PROGRAM ModbusRTU_Master
VAR
	ModbusRtuMaster	: ModbusRtuMasterV2_Generic;
	Timeout			: TIME:=T#1S;
	Data_01			: WORD;
	Data_02			: WORD;
	Data_03			: ARRAY[1..10] OF WORD;
	Data_04			: ARRAY[1..10] OF WORD;	
	Data_05			: WORD:=1;	 
	Data_06			: WORD:=666;
	Data_07			: DWORD:=3;
	Data_08			: ARRAY[1..100] OF WORD:=[100(1)];
	
	step		: INT;
	Start		: BOOL;
	i			: INT;
	ErrMsg_01: Tc2_ModbusRTU.MODBUS_ERRORS;
	ErrMsg_02: Tc2_ModbusRTU.MODBUS_ERRORS;
	ErrMsg_03: Tc2_ModbusRTU.MODBUS_ERRORS;
	ErrMsg_04: Tc2_ModbusRTU.MODBUS_ERRORS;
	ErrMsg_05: Tc2_ModbusRTU.MODBUS_ERRORS;
	ErrMsg_06: Tc2_ModbusRTU.MODBUS_ERRORS;
	ErrMsg_07: Tc2_ModbusRTU.MODBUS_ERRORS;
	ErrMsg_08: Tc2_ModbusRTU.MODBUS_ERRORS;
	ErrCount_01: INT;
	ErrCount_02: INT;
	ErrCount_03: INT;
	ErrCount_04: INT;
	ErrCount_05: INT;
	ErrCount_06: INT;
	ErrCount_07: INT;
	ErrCount_08: INT;
	ResetErrCount: BOOL;
	Counter: INT;
END_VAR

IF ResetErrCount THEN
	ErrCount_01:=0;
	ErrCount_02:=0;
	ErrCount_03:=0;
	ErrCount_04:=0;
	ErrCount_05:=0;
	ErrCount_06:=0;
	ErrCount_07:=0;
	ErrCount_08:=0;
	ResetErrCount:=FALSE;
END_IF
CASE step OF 
0: 
IF Start THEN
	step:=8;
	Counter:=Counter+1;	
//	Start:=FALSE;
END_IF
1:
// 读取线圈，对应Modsim中 01:Coil Status
	ModbusRtuMaster.ReadCoils(
		UnitID:=1 , 
		Quantity:=10 , 
		MBAddr:=0 , 	// 起始地址0，对应Modsim中地址00001——00010
		cbLength:=SIZEOF(Data_01) , // 读取10个bit，放在一个word中，占用2个字节 , 
		pMemoryAddr:=ADR(Data_01) , 
		AuxQuantity:= , 
		AuxMBAddr:= , 
		AuxcbLength:= , 
		pAuxMemoryAddr:= , 
		Execute:=TRUE , 
		Timeout:=Timeout , 
		RxBuffer:=RxBuffer , 
		TxBuffer:=TxBuffer , 
		BUSY=> , 
		Error=> , 
		ErrorId=> , 
		cbRead=> );
	IF NOT ModbusRtuMaster.BUSY THEN
		ModbusRtuMaster.ReadCoils(	Execute:=FALSE , RxBuffer:=RxBuffer , TxBuffer:=TxBuffer );
		step:=step+1;
		IF ModbusRtuMaster.Error THEN
			ErrMsg_01:=ModbusRtuMaster.ErrorId;
			ErrCount_01:=ErrCount_01+1;
		END_IF
	END_IF
2:
// 读取输入状态，对应Modsim中 02:Input Status
	ModbusRtuMaster.ReadInputStatus(
	UnitID:=1 , 
	Quantity:=10 , 	// 读取10个bit状态
	MBAddr:=0 , 	// 起始地址0，对应Modsim中地址10001——10010
	cbLength:=SIZEOF(Data_02) , // 读取10个bit，放在一个word中，占用2个字节
	pMemoryAddr:=ADR(Data_02) , 
	AuxQuantity:= , 
	AuxMBAddr:= , 
	AuxcbLength:= , 
	pAuxMemoryAddr:= , 
	Execute:=TRUE , 
	Timeout:=Timeout , 
	RxBuffer:=RxBuffer , 
	TxBuffer:=TxBuffer , 
	BUSY=> , 
	Error=> , 
	ErrorId=> , 
	cbRead=> );
	IF NOT ModbusRtuMaster.BUSY THEN
		ModbusRtuMaster.ReadInputStatus(	Execute:=FALSE , RxBuffer:=RxBuffer , TxBuffer:=TxBuffer );
		step:=step+1;
		IF ModbusRtuMaster.Error THEN
			ErrMsg_02:=ModbusRtuMaster.ErrorId;
			ErrCount_02:=ErrCount_02+1;
		END_IF
	END_IF
3:
// 读取保持寄存器，对应Modsim中 03:Holding Registers
	ModbusRtuMaster.ReadRegs(
	UnitID:=1 , 
	Quantity:=10 , 	// 读取10个寄存器数值，20个BYTE
	MBAddr:=0 , 	// 起始地址，0对应Modsim中地址40001——40010
	cbLength:=SIZEOF(Data_03) , // 读取10个寄存器，放在一个数组中，占用20个字节
	pMemoryAddr:=ADR(Data_03) , 
	AuxQuantity:= , 
	AuxMBAddr:= , 
	AuxcbLength:= , 
	pAuxMemoryAddr:= , 
	Execute:=TRUE , 
	Timeout:=Timeout , 
	RxBuffer:=RxBuffer , 
	TxBuffer:=TxBuffer , 
	BUSY=> , 
	Error=> , 
	ErrorId=> , 
	cbRead=> );
	IF NOT ModbusRtuMaster.BUSY THEN
		ModbusRtuMaster.ReadRegs(	Execute:=FALSE , RxBuffer:=RxBuffer , TxBuffer:=TxBuffer );
		step:=step+1;
		IF ModbusRtuMaster.Error THEN
			ErrMsg_03:=ModbusRtuMaster.ErrorId;
			ErrCount_03:=ErrCount_03+1;
		END_IF
	END_IF
4:
// 读取输入寄存器，对应Modsim中 04:Input Registers
	ModbusRtuMaster.ReadInputRegs(
	UnitID:=1 , 
	Quantity:=10 , 	// 读取10个寄存器数值，20个BYTE
	MBAddr:=0 , 	// 起始地址，0对应Modsim中地址30001——30010
	cbLength:=SIZEOF(Data_04) , // 读取10个寄存器，放在一个数组中，占用20个字节
	pMemoryAddr:=ADR(Data_04) , 
	AuxQuantity:= , 
	AuxMBAddr:= , 
	AuxcbLength:= , 
	pAuxMemoryAddr:= , 
	Execute:=TRUE , 
	Timeout:=Timeout , 
	RxBuffer:=RxBuffer , 
	TxBuffer:=TxBuffer , 
	BUSY=> , 
	Error=> , 
	ErrorId=> , 
	cbRead=> );
	IF NOT ModbusRtuMaster.BUSY THEN
		ModbusRtuMaster.ReadInputRegs(	Execute:=FALSE , RxBuffer:=RxBuffer , TxBuffer:=TxBuffer );
		step:=step+1;
		IF ModbusRtuMaster.Error THEN
			ErrMsg_04:=ModbusRtuMaster.ErrorId;
			ErrCount_04:=ErrCount_04+1;
		END_IF
		Data_05.0:=NOT Data_05.0;
	END_IF
5:
// 写入单个线圈Force Single Coil，对应Modsim中 01:Coil Status
	ModbusRtuMaster.WriteSingleCoil(
	UnitID:=1 , 
	Quantity:=1 , 	// 写入1个bit
	MBAddr:=50 , 	// 起始地址，50对应Modsim中地址00051
	cbLength:=SIZEOF(Data_05) , 
	pMemoryAddr:=ADR(Data_05) , 
	AuxQuantity:= , 
	AuxMBAddr:= , 
	AuxcbLength:= , 
	pAuxMemoryAddr:= , 
	Execute:=TRUE , 
	Timeout:=Timeout , 
	RxBuffer:=RxBuffer , 
	TxBuffer:=TxBuffer , 
	BUSY=> , 
	Error=> , 
	ErrorId=> , 
	cbRead=> );
	IF NOT ModbusRtuMaster.BUSY THEN
		ModbusRtuMaster.WriteSingleCoil(	Execute:=FALSE , RxBuffer:=RxBuffer , TxBuffer:=TxBuffer );
		step:=step+1;
		IF ModbusRtuMaster.Error THEN
			ErrMsg_05:=ModbusRtuMaster.ErrorId;
			ErrCount_05:=ErrCount_05+1;
		END_IF
		Data_06:=Data_06+1;
	END_IF
6:
// 写入单个寄存器Preset Single Register，对应Modsim中 03:Holding Registers
	ModbusRtuMaster.WriteSingleRegister(
	UnitID:=1 , 
	Quantity:=1 , 	// 写入1个寄存器，2个Byte
	MBAddr:=50 , 	// 起始地址，50对应Modsim中地址40051
	cbLength:=SIZEOF(Data_06) , 
	pMemoryAddr:=ADR(Data_06) , 
	AuxQuantity:= , 
	AuxMBAddr:= , 
	AuxcbLength:= , 
	pAuxMemoryAddr:= , 
	Execute:=TRUE , 
	Timeout:=Timeout , 
	RxBuffer:=RxBuffer , 
	TxBuffer:=TxBuffer , 
	BUSY=> , 
	Error=> , 
	ErrorId=> , 
	cbRead=> );
	IF NOT ModbusRtuMaster.BUSY THEN
		ModbusRtuMaster.WriteSingleRegister(	Execute:=FALSE , RxBuffer:=RxBuffer , TxBuffer:=TxBuffer );
		step:=step+1;
		IF ModbusRtuMaster.Error THEN
			ErrMsg_06:=ModbusRtuMaster.ErrorId;
			ErrCount_06:=ErrCount_06+1;
		END_IF
		Data_07:=ROL(Data_07,1);
	END_IF
7:
// 写入多个线圈Force Multiple Coils，对应Modsim中 01:Coil Status
	ModbusRtuMaster.WriteMultipleCoils(
	UnitID:=1 , 
	Quantity:=20 , 	// 写入20个bit
	MBAddr:=80 , 	// 起始地址，80对应Modsim中地址00081——00100
	cbLength:=SIZEOF(Data_07) , 	// 数据来自一个DWORD
	pMemoryAddr:=ADR(Data_07) , 
	AuxQuantity:= , 
	AuxMBAddr:= , 
	AuxcbLength:= , 
	pAuxMemoryAddr:= , 
	Execute:=TRUE , 
	Timeout:=Timeout , 
	RxBuffer:=RxBuffer , 
	TxBuffer:=TxBuffer , 
	BUSY=> , 
	Error=> , 
	ErrorId=> , 
	cbRead=> );
	IF NOT ModbusRtuMaster.BUSY THEN
		ModbusRtuMaster.WriteMultipleCoils(	Execute:=FALSE , RxBuffer:=RxBuffer , TxBuffer:=TxBuffer );
		step:=step+1;
		IF ModbusRtuMaster.Error THEN
			ErrMsg_07:=ModbusRtuMaster.ErrorId;
			ErrCount_07:=ErrCount_07+1;
		END_IF
		FOR i:=1 TO 20 DO
			Data_08[i]:=Data_08[i]+1;
		END_FOR		
	END_IF
8:
// 写入多个寄存器Preset Multiple Registers，对应Modsim中 03:Holding Registers
	ModbusRtuMaster.WriteRegs(
	UnitID:=1 , 
	Quantity:=20 , 	// 写入20个寄存器，40个Byte
	MBAddr:=80 , 	// 起始地址，80对应Modsim中地址40081——40100
	cbLength:=SIZEOF(Data_08) , // 要写入的数据
	pMemoryAddr:=ADR(Data_08) , 
	AuxQuantity:= , 
	AuxMBAddr:= , 
	AuxcbLength:= , 
	pAuxMemoryAddr:= , 
	Execute:=TRUE , 
	Timeout:=Timeout , 
	RxBuffer:=RxBuffer , 
	TxBuffer:=TxBuffer , 
	BUSY=> , 
	Error=> , 
	ErrorId=> , 
	cbRead=> );
	IF NOT ModbusRtuMaster.BUSY THEN
		ModbusRtuMaster.WriteRegs(	Execute:=FALSE , RxBuffer:=RxBuffer , TxBuffer:=TxBuffer );
		step:=0;
		IF ModbusRtuMaster.Error THEN
			ErrMsg_08:=ModbusRtuMaster.ErrorId;
			ErrCount_08:=ErrCount_08+1;
		END_IF
	END_IF
END_CASE

END_PROGRAM
